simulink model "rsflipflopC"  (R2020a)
settings: Solver=ode45  StartTime=0.0  StopTime=Inf  FixedStep=1  RelTol=1e-3  EnableMultiTasking=on

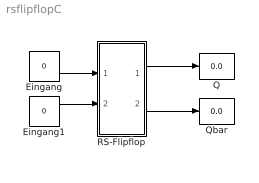
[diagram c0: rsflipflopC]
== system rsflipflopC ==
  note: .
  Eingang : Constant  Value=0  OutDataTypeStr=double
  Eingang1 : Constant  Value=0  OutDataTypeStr=double
  Q : Display
  Qbar : Display
  RS-Flipflop : Subsystem  mask(SRFlipFlop){initial_condition=0}
      mask prompts: initial_condition "Initial condition (state of Q):"
      mask help: S-R Flip-Flop Block
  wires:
  Eingang/1 -> RS-Flipflop/1(S)
  Eingang1/1 -> RS-Flipflop/2(R)
  RS-Flipflop/1(Q) -> Q/1
  RS-Flipflop/2(!Q) -> Qbar/1

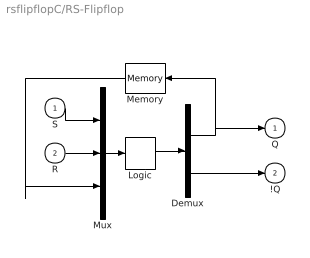
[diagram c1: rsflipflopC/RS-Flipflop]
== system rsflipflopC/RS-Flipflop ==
  note: .
  S : Inport
  R : Inport  Port=2
  Demux : Demux  Outputs=2
  Logic : CombinatorialLogic  TruthTable=[0 1;1 0;0 1;0 1;1 0;1 0;0 0;0 0]
  Memory : Memory  InitialCondition=initial_condition  InheritSampleTime=on
  Mux : Mux  Inputs=3
  Q : Outport  InitialOutput=0
  !Q : Outport  Port=2  InitialOutput=1
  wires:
  Memory/1 -> Mux/3
  Mux/1 -> Logic/1
  Logic/1 -> Demux/1
  Demux/2 -> !Q/1
  Demux/1 -> Q/1, Memory/1
  S/1 -> Mux/1
  R/1 -> Mux/2
